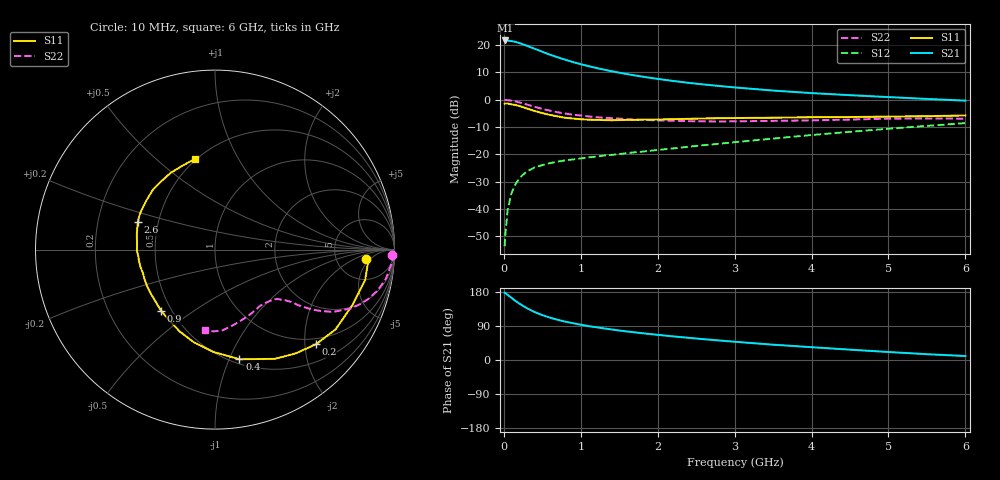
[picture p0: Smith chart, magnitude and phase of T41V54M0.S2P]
! Infineon Technologies  Discrete & RF Semiconductors
! BFR182T
! Si NPN RF Bipolar Junction Transistor in SC75
! VCE = 1.5 V  IC = 4 mA
! Common Emitter S-Parameters:  October  1999
# GHz  S  MA  R  50
!  f  S11  S21  S12  S22
! GHz  MAG  ANG  MAG  ANG  MAG  ANG  MAG  ANG
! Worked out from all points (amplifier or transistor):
!   36 points, 10 MHz to 6 GHz, reference 50 ohm
!   highest |S21| = 21.7 dB at 20 MHz (marker M1)
!   |S21| within 3 dB of that: start of sweep to 397.1 MHz
!   unconditionally stable (mu >= 1): 1.474 GHz to 4.179 GHz
!   at 250 MHz: K = 0.24, MSG = 23.8 dB, |S12| = -27.4 dB
!   at 1.4 GHz: K = 0.98, MSG = 15.3 dB, |S12| = -20.2 dB
!   at 6 GHz: K = 0.85, MSG = 4.1 dB, |S12| = -8.5 dB
!   S11 on the Smith chart (normalised r, x): 10 MHz: 11, -4; 200 MHz: 0.86, -2.24; 400 MHz: 0.54, -1.09; 900 MHz: 0.44, -0.38; 2.6 GHz: 0.38, +0.15; 6 GHz: 0.49, +0.68
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0.01  0.8448 -3.4  12.18 177.7  0.0021 80.4  0.9853 -1.7
0.02  0.8576 -3.4  12.19 176.9  0.0035 97.8  0.994 -2.0
0.05  0.8537 -11.5  12.16 171.7  0.0097 87.2  0.9847 -5.0
0.1  0.8257 -22.0  11.85 164.0  0.0196 81.2  0.966 -9.7
0.15  0.8056 -33.5  11.48 156.1  0.0285 73.5  0.9345 -14.1
0.2  0.7709 -43.2  10.97 149.1  0.0364 69.3  0.8984 -17.8
0.25  0.7319 -52.3  10.35 142.7  0.0427 64.5  0.8572 -21.1
0.3  0.6935 -61.4  9.746 136.7  0.049 61.3  0.8197 -23.7
0.4  0.6257 -77.4  8.601 126.5  0.0579 55.7  0.744 -27.8
0.5  0.571 -90.7  7.57 118.5  0.0639 52.8  0.6824 -30.1
0.6  0.5293 -103.0  6.694 111.7  0.0694 50.5  0.6327 -31.8
0.7  0.4967 -113.4  5.995 106.1  0.074 49.1  0.5917 -32.8
0.8  0.4689 -122.9  5.408 101.1  0.0781 48.3  0.5598 -33.7
0.9  0.4547 -131.2  4.9 97.0  0.0812 48.2  0.5333 -34.1
1.1  0.4333 -145.8  4.136 89.4  0.0884 49.0  0.4969 -35.2
1.6  0.4285 -171.6  2.954 75.3  0.106 51.8  0.4425 -38.4
2.2  0.4429 169.7  2.215 62.3  0.1292 55.9  0.4143 -44.7
2.6  0.4563 160.5  1.908 54.9  0.148 57.7  0.4037 -49.7
3.5  0.4704 144.0  1.477 40.4  0.1954 59.1  0.4117 -62.3
4.5  0.4841 128.6  1.216 27.3  0.2598 57.3  0.4353 -77.4
5.5  0.5021 110.9  1.038 15.3  0.334 52.9  0.4559 -91.2
6  0.5167 102.4  0.965 10.5  0.3744 49.6  0.4524 -97.3
